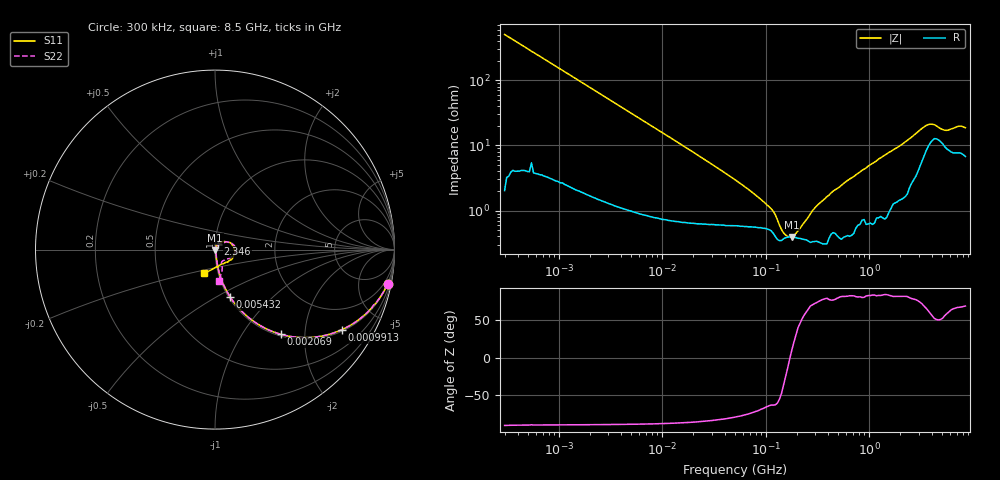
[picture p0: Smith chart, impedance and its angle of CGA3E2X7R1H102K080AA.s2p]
! S-parameter Generated by TDK Corporation
! Copyright(C) 2015 TDK Corporation.
! All Rights Reserved.
! TDK P/N: CGA3E2X7R1H102K080AA (Multilayer Ceramic Chip Capacitors)
! Property: C=1nF
! Size(LxWxT): 1.6x0.8x0.8mm, 0.063x0.031x0.031inches
! Model Type: s2p (Touchstone File Format Version 1.0)
! Frequency: DC=Yes Start=0.3MHz Stop=8500MHz 225points Log-sweep
! Note:
! Model Generated on Jun. 23, 2015
! Hash(MD5):
! Port Assignments:
!  1 ---| |--- 2
! Applicable Conditions:
!  Temperature = 25 degC
!  DC Bias Voltage = 0 V
!  Small Signal Operation
! Terms and conditions regarding TDK Simulation Models
! (1)This simulation model is being provided solely for informational purposes. Please refer to the specifications of the products in terms of detailed characteristics of such products.
! (2)In no event shall TDK Corporation of any of its subsidiaries be liable for any loss or damage arising, directly or indirectly,
!  From any information contained in this simulation model, including, but not limited to loss or damages arising from any inaccuracies, omissions or errors in connection with such information.
! (3)Any and all copyrights on this simulation model are owned by TDK Corporation.
!  Duplication or redistribution of this simulation model without prior written permission from TDK Corporation is prohibited.
! (4)This simulation model is subject to any modification or change without any prior notice.
! (5)Neither TDK Corporation nor any of its subsidiaries shall make any warranty, express or implied,
!  Including but not limited to the correctness, implied warranties of merchantability and fitness for a particular purpose with respect to this simulation models.
! (6)The use of this simulation model shall be deemed to have consented to the terms and conditions hereof.
# MHz S MA R 50
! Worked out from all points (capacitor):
!   224 points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, 300 kHz to 8.5 GHz, reference 50 ohm
!   read as one part in series: C = 1.04 nF near 314.1 kHz
!   lowest |Z| = 392 mohm at 178.8 MHz (marker M1)
!   series resonance near 171.5 MHz, so ESL is about 830 pH
!   S11 on the Smith chart (normalised r, x): 300 kHz: 1, -10; 991.3 kHz: 1.06, -3.12; 2.069 MHz: 1.03, -1.51; 5.432 MHz: 1.02, -0.58; 2.346 GHz: 1.03, +0.07; 8.5 GHz: 0.86, -0.23
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0.3  0.9808 -11.3  0.1934 78.5  0.1935 78.8  0.9808 -11.2
0.9913414  0.8353 -32.3  0.5357 56.7  0.5343 56.8  0.8351 -32.4
1.72111  0.665 -47.2  0.7353 41.6  0.7337 41.8  0.6646 -47.2
2.068572  0.5969 -52.2  0.7915 36.5  0.7898 36.7  0.5965 -52.2
5.431819  0.2767 -72.3  0.9535 15.9  0.9518 16.1  0.2765 -72.3
9.430415  0.1645 -78.2  0.9801 9.3  0.9785 9.5  0.1643 -78.2
51.67171  0.03023 -78.9  0.9942 1.4  0.9929 1.6  0.03138 -77.7
178.7805  0.004788 -71.9  0.9955 -0.5  0.9943 -0.3  0.008312 -63.6
270.4017  0.001044 -53.9  0.9954 -1.1  0.9941 -0.9  0.00257 -45.5
283.1228  0.0002995 -34.7  0.9953 -1.2  0.9939 -1.0  0.002688 -33.9
310.3886  0.0007554 79.0  0.9949 -1.4  0.9935 -1.2  0.001831 -15.4
340.2802  0.0009098 92.1  0.9947 -1.6  0.9933 -1.3  0.001178 40.3
373.0505  0.0007577 83.2  0.9946 -1.7  0.9933 -1.5  0.00207 81.6
448.3627  0.004361 41.1  0.9943 -2.1  0.993 -1.9  0.004382 52.3
514.6664  0.00499 68.8  0.9942 -2.5  0.9929 -2.2  0.003656 74.9
710.042  0.005417 75.3  0.9927 -3.5  0.9916 -3.2  0.01026 79.0
893.5346  0.01396 55.7  0.9924 -4.3  0.9912 -4.1  0.01287 58.0
1551.304  0.02239 67.8  0.9869 -7.7  0.9858 -7.5  0.02435 69.1
2346.313  0.03602 62.1  0.977 -11.7  0.9755 -11.4  0.04143 53.9
3548.748  0.09477 23.9  0.917 -17.4  0.9157 -17.1  0.09895 21.0
6161.135  0.09386 -47.6  0.9158 -21.9  0.917 -21.5  0.07739 -59.9
8500  0.1446 -114.0  0.9081 -30.8  0.9076 -30.0  0.1764 -82.9
